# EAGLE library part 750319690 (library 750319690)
WE-PPTI Push-Pull Transformer TOR6/3/3 SMT; Ui = 12V; Uo1 = 5V/0.7A; f = 400-600kHz Source: Datasheet
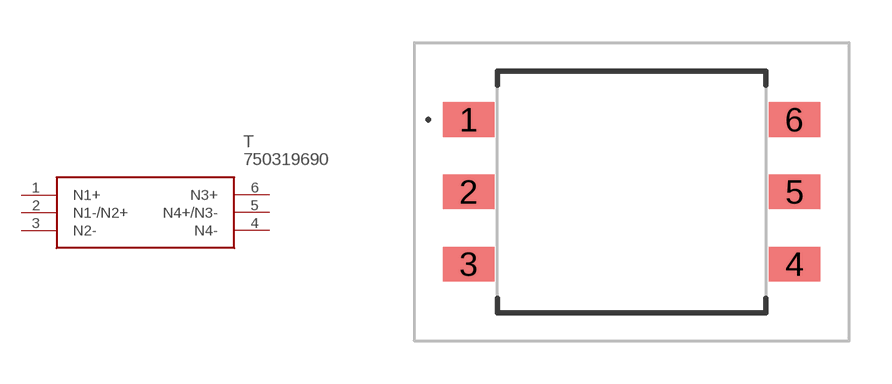
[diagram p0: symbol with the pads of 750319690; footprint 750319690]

Designator prefix T

## 750319690 (Description: WE-PPTI Push-Pull Transformer TOR6/3/3 SMT; Ui = 12V; Uo1 = 5V/0.7A; f = 400-600kHz; Height: 5.5mm; Manufacturer_Name: Wurth Elektronik; Manufacturer_Part_Number: 750319690; Mouser_Part_Number: 710-750319690; Mouser_Price-Stock: https://www.mouser.co.uk/ProductDetail/Wurth-Elektronik/750319690?qs=1Kr7Jg1SGW%2Fxuc9sXU4Xvg%3D%3D)  [750319690]
1  N1+
2  N1-/N2+
3  N2-
4  N4-
5  N4+/N3-
6  N3+

## Footprint 750319690 (pad centres in mm)
750319690-2
smd 1.82 x 1.22: 1 -5.725,2.54; 2 -5.725,0; 3 -5.725,-2.54; 4 5.725,-2.54; 5 5.725,0; 6 5.725,2.54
